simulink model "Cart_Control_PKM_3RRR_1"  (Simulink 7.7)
settings: Solver=FixedStepDiscrete  SolverMode=SingleTasking  StartTime=0  StopTime=6  FixedStep=dt  RelTol=1e-3  SampleTimeConstraint=Specified
InitFcn:
  | % Sampling Times %
  | dt0=0.001; dt1=0.01; samples=10;
  | D2R=pi/180;
undefined symbols (not defined in the file or in its folder): DiscIntNeverNeededParam, Volts
libraries: simulink_extras x4, speedgoatlib_IO311 x3, simulink x3, speedgoatlib x2, xpclib x1

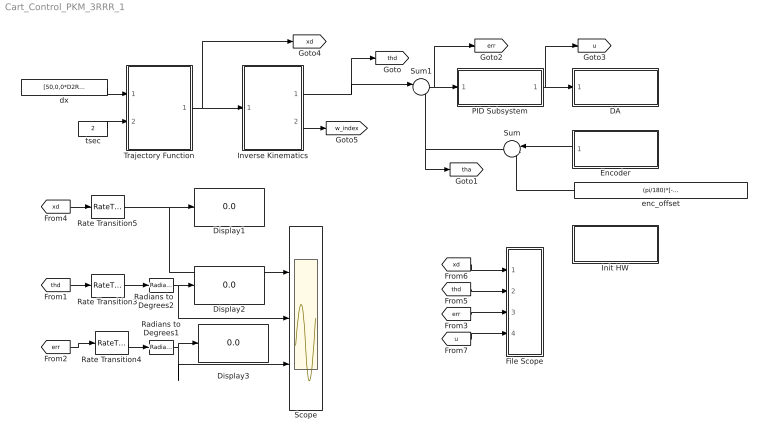
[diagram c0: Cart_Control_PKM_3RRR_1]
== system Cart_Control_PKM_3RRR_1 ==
  DA : Subsystem  TreatAsAtomicUnit=on
  Display1 : Display
  Display2 : Display
  Display3 : Display
  Encoder : Subsystem  TreatAsAtomicUnit=on
  File Scope : Subsystem
  Init HW : Subsystem  TreatAsAtomicUnit=on
  Inverse Kinematics : Stateflow chart  TreatAsAtomicUnit=on
  PID Subsystem : Subsystem  TreatAsAtomicUnit=on
  Radians to Degrees1 : simulink_extras/Transformations/Radians to Degrees  SystemSampleTime=-1
  Radians to Degrees2 : simulink_extras/Transformations/Radians to Degrees  SystemSampleTime=-1
  Rate Transition3 : RateTransition  OutPortSampleTime=dt1
  Rate Transition4 : RateTransition  OutPortSampleTime=dt1
  Rate Transition5 : RateTransition  OutPortSampleTime=dt1
  Scope : Scope  NumInputPorts=3
  Sum : Sum  Inputs=|++
  Sum1 : Sum  Inputs=|+-
  Trajectory Function : Stateflow chart  TreatAsAtomicUnit=on
  dx : Constant  Value=[50,0,0*D2R]'  SampleTime=dt0
  enc_offset : Constant  Value=(pi/180)*[-144.9004,-24.9004,95.0996]'
  tsec : Constant  Value=2  SampleTime=dt0
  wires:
  Sum1/1 -> PID Subsystem/1(In1), [err]
  PID Subsystem/1(Out1) -> [u], DA/1(In1)
  Encoder/1(Out1) -> Sum/1
  enc_offset/1 -> Sum/2
  Sum/1 -> Sum1/2, [tha]
  [xd] -> File Scope/1(xd)
  [thd] -> File Scope/2(thd)
  [err] -> File Scope/3(err)
  [u] -> File Scope/4(u)
  dx/1 -> Trajectory Function/1(dx)
  tsec/1 -> Trajectory Function/2(tsec)
  Trajectory Function/1(xd) -> [xd], Inverse Kinematics/1(xd)
  Inverse Kinematics/1(thd) -> Sum1/1, [thd]
  [thd] -> Rate Transition3/1
  [err] -> Rate Transition4/1
  [xd] -> Rate Transition5/1
  Rate Transition5/1 -> Display1/1, Scope/1
  Rate Transition3/1 -> Radians to Degrees2/1
  Rate Transition4/1 -> Radians to Degrees1/1
  Radians to Degrees2/1 -> Display2/1, Scope/2
  Radians to Degrees1/1 -> Display3/1, Scope/3
  Inverse Kinematics/2(w_index) -> [w_index]

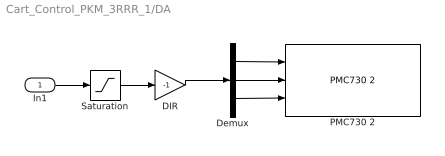
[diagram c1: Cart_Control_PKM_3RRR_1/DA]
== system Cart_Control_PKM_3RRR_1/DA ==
  In1 : Inport
  DIR : Gain  Gain=-1
  Demux : Demux  Outputs=3
  PMC730 2 : speedgoatlib/IO101/PMC730 2  id=1  channel=[1,2,3]  reset=[1,1,1]  initValue=[0,0,0]  ts=dt0  pciSlot=-1
  Saturation : Saturate  UpperLimit=10  LowerLimit=-10
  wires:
  In1/1 -> Saturation/1
  Saturation/1 -> DIR/1
  DIR/1 -> Demux/1
  Demux/1 -> PMC730 2/1
  Demux/2 -> PMC730 2/2
  Demux/3 -> PMC730 2/3

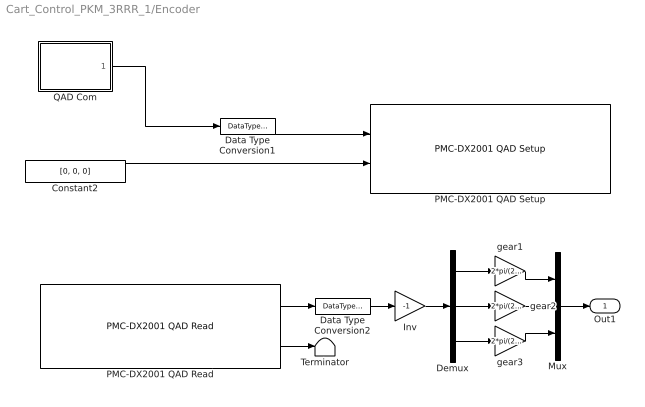
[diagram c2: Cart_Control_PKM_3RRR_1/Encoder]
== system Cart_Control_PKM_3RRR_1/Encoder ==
  Constant2 : Constant  Value=[0, 0, 0]  OutDataTypeStr=Inherit: Inherit via back propagation
  Data Type Conversion1 : DataTypeConversion  OutDataTypeStr=uint8
  Data Type Conversion2 : DataTypeConversion  OutDataTypeStr=double
  Demux : Demux  Outputs=3
  Inv : Gain  Gain=-1
  Mux : Mux  Inputs=3
  PMC-DX2001 QAD Read : speedgoatlib_IO311/PMC-DX2001 QAD Read  id=1  chan=[1, 2, 3]  pciSlot=-1  ts=dt0
  PMC-DX2001 QAD Setup : speedgoatlib_IO311/PMC-DX2001 QAD Setup  id=1  chan=Channel 3 setup  steps1=2000  steps2=2000  steps3=2000  quadrature1=4x  quadrature2=4x  quadrature3=4x  index1=Ignore index input  index2=Ignore index input  index3=Ignore index input  special1=Disabled (cycling counter)  special2=Disabled (cycling counter)  special3=Disabled (cycling counter)  debounce=0  pciSlot=-1  ts=dt0
  QAD Com : Stateflow chart  TreatAsAtomicUnit=on
  Terminator : Terminator
  gear1 : Gain  Gain=2*pi/(23*2000)
  gear2 : Gain  Gain=2*pi/(23*2000)
  gear3 : Gain  Gain=2*pi/(23*2000)
  Out1 : Outport
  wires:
  Constant2/1 -> PMC-DX2001 QAD Setup/2
  PMC-DX2001 QAD Read/2 -> Terminator/1
  PMC-DX2001 QAD Read/1 -> Data Type Conversion2/1
  QAD Com/1(y) -> Data Type Conversion1/1
  Data Type Conversion1/1 -> PMC-DX2001 QAD Setup/1
  Data Type Conversion2/1 -> Inv/1
  Mux/1 -> Out1/1
  Demux/1 -> gear1/1
  gear1/1 -> Mux/1
  Demux/2 -> gear2/1
  gear2/1 -> Mux/2
  Inv/1 -> Demux/1
  Demux/3 -> gear3/1
  gear3/1 -> Mux/3

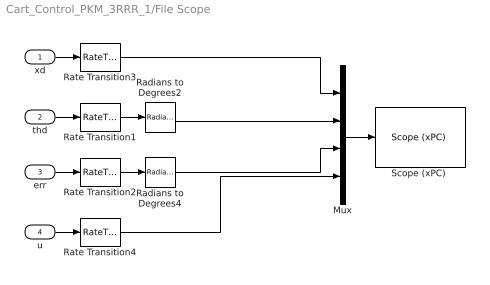
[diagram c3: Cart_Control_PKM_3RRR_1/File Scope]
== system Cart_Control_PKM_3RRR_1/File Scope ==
  xd : Inport
  thd : Inport  Port=2
  err : Inport  Port=3
  u : Inport  Port=4
  Mux : Mux
  Radians to Degrees2 : simulink_extras/Transformations/Radians to Degrees  SystemSampleTime=-1
  Radians to Degrees4 : simulink_extras/Transformations/Radians to Degrees  SystemSampleTime=-1
  Rate Transition{1..4} (4 alike) : RateTransition  OutPortSampleTime=dt1
  "Scope (xPC) " : xpclib/Misc./Scope (xPC)   SystemSampleTime=-1  scopeno=1  scopetype=File  autostart=on  viewmode=Graphical redraw  formatstr='%15.6f'  grid=on  ylimits=[0,0]  nosamples=100  noprepostsamples=0  interleave=1  triggermode=FreeRun  triggersignal=1  triggerlevel=0.0  triggerslope=Either  triggerscope=1  triggersample=0  filename=step2.dat  mode=Lazy  writesize=512  autorestart=on  dynamicfilemode=off  maxwritefilesize=512*1024^2
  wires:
  Radians to Degrees2/1 -> Mux/2
  Radians to Degrees4/1 -> Mux/3
  Rate Transition1/1 -> Radians to Degrees2/1
  Rate Transition2/1 -> Radians to Degrees4/1
  thd/1 -> Rate Transition1/1
  err/1 -> Rate Transition2/1
  Rate Transition3/1 -> Mux/1
  xd/1 -> Rate Transition3/1
  u/1 -> Rate Transition4/1
  Mux/1 -> "Scope (xPC) "/1
  Rate Transition4/1 -> Mux/4

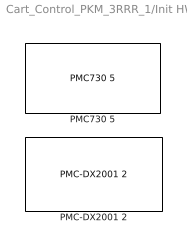
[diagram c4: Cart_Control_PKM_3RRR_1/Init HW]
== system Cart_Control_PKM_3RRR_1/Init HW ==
  PMC-DX2001 2 : speedgoatlib_IO311/PMC-DX2001 2  id=1  fpga1=IO311_3PWM_3CAP_3QAD_INT.fpga  fpga2=PWM_Triangle_DX501.fpga  fpga3=PWM_Triangle_DX501.fpga  fpga4=PWM_Triangle_DX501.fpga  fpga5=PWM_Triangle_DX501.fpga  fpga6=PWM_Triangle_DX501.fpga  fpga7=PWM_Triangle_DX501.fpga  fpga8=PWM_Triangle_DX501.fpga  fpga9=PWM_Triangle_DX501.fpga  fpga10=PWM_Triangle_DX501.fpga  group=Module setup  pciSlot=-1  lowerDirection=[ones(1,5), zeros(1, 7), ones(1, 1), ones(1, 3)]  lowerReset=[1]  lowerValue=[0]  upperDirection=[ones(1, 8), zeros(1, 8)]  upperReset=[1]  upperValue=[0]
  PMC730 5 : speedgoatlib/IO101/PMC730 5  id=1  group=Analog output setup  pciSlot=-1  adStartChannel=1  adNumChannel=1  adCoupling=Single-ended  adRange=-10 .. 10 Volts  adAcqMode=Standard  daChannel=[1,2, 3]  daReset=[1,1, 1]  daInitValue=[0,0,0]  diChannel=[1]  diDebounce=[0]  doChannel=[1]  doReset=[1]  doInitValue=[0]

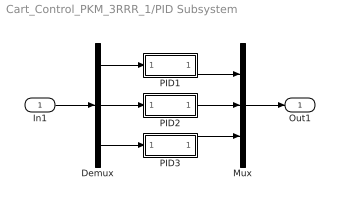
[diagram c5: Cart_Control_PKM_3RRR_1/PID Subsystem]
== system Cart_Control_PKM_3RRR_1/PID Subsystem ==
  In1 : Inport
  Demux : Demux  Outputs=3
  Mux : Mux  Inputs=3
  PID1 : Subsystem
  PID2 : Subsystem
  PID3 : Subsystem
  Out1 : Outport
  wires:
  In1/1 -> Demux/1
  Demux/1 -> PID1/1(In1)
  PID1/1(Out1) -> Mux/1
  Demux/2 -> PID2/1(In1)
  PID2/1(Out1) -> Mux/2
  Mux/1 -> Out1/1
  Demux/3 -> PID3/1(In1)
  PID3/1(Out1) -> Mux/3

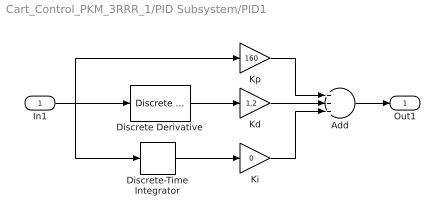
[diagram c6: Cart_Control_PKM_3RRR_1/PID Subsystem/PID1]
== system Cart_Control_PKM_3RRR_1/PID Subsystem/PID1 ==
  In1 : Inport
  Add : Sum  Inputs=+++
  Discrete Derivative : simulink/Discrete/Discrete Derivative  SystemSampleTime=-1  gainval=1.0  ICPrevScaledInput=0.0  OutMin=[]  OutMax=[]  OutDataType=fixdt(1, 16)  OutScaling=2^-10  DoSatur=off
  Discrete-Time Integrator : DiscreteIntegrator  SampleTime=dt0  ICPrevOutput=DiscIntNeverNeededParam  ICPrevScaledInput=DiscIntNeverNeededParam
  Kd : Gain  Gain=1.2
  Ki : Gain  Gain=0
  Kp : Gain  Gain=160
  Out1 : Outport
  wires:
  Discrete-Time Integrator/1 -> Ki/1
  Kp/1 -> Add/1
  Kd/1 -> Add/2
  Ki/1 -> Add/3
  Discrete Derivative/1 -> Kd/1
  Add/1 -> Out1/1
  In1/1 -> Kp/1, Discrete Derivative/1, Discrete-Time Integrator/1

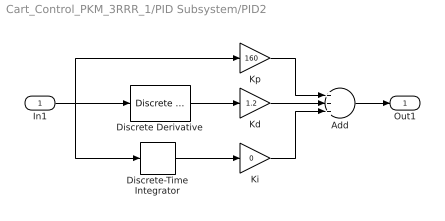
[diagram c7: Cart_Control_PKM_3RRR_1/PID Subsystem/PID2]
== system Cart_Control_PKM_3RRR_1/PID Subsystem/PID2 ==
  In1 : Inport
  Add : Sum  Inputs=+++
  Discrete Derivative : simulink/Discrete/Discrete Derivative  SystemSampleTime=-1  gainval=1.0  ICPrevScaledInput=0.0  OutMin=[]  OutMax=[]  OutDataType=fixdt(1, 16)  OutScaling=2^-10  DoSatur=off
  Discrete-Time Integrator : DiscreteIntegrator  SampleTime=dt0  ICPrevOutput=DiscIntNeverNeededParam  ICPrevScaledInput=DiscIntNeverNeededParam
  Kd : Gain  Gain=1.2
  Ki : Gain  Gain=0
  Kp : Gain  Gain=160
  Out1 : Outport
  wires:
  Discrete-Time Integrator/1 -> Ki/1
  Kp/1 -> Add/1
  Kd/1 -> Add/2
  Ki/1 -> Add/3
  Discrete Derivative/1 -> Kd/1
  Add/1 -> Out1/1
  In1/1 -> Kp/1, Discrete Derivative/1, Discrete-Time Integrator/1

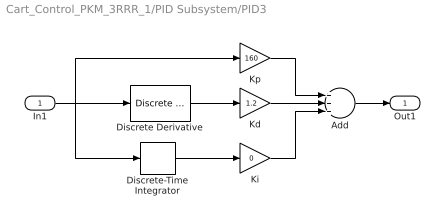
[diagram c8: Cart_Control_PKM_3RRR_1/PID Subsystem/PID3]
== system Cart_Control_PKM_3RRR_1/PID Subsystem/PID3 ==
  In1 : Inport
  Add : Sum  Inputs=+++
  Discrete Derivative : simulink/Discrete/Discrete Derivative  SystemSampleTime=-1  gainval=1.0  ICPrevScaledInput=0.0  OutMin=[]  OutMax=[]  OutDataType=fixdt(1, 16)  OutScaling=2^-10  DoSatur=off
  Discrete-Time Integrator : DiscreteIntegrator  SampleTime=dt0  ICPrevOutput=DiscIntNeverNeededParam  ICPrevScaledInput=DiscIntNeverNeededParam
  Kd : Gain  Gain=1.2
  Ki : Gain  Gain=0
  Kp : Gain  Gain=160
  Out1 : Outport
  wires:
  Discrete-Time Integrator/1 -> Ki/1
  Kp/1 -> Add/1
  Kd/1 -> Add/2
  Ki/1 -> Add/3
  Discrete Derivative/1 -> Kd/1
  Add/1 -> Out1/1
  In1/1 -> Kp/1, Discrete Derivative/1, Discrete-Time Integrator/1

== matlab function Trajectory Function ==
function xd = fcn(dx, tsec)

persistent index xd_p

MAX_CH=3;       % 3 Actuators %
dt=0.001;       % Step time is 10 msec %

% Initializing Variables %
if isempty(index), index=0; end
if isempty(xd_p), xd_p=zeros(MAX_CH,1); end
xd=zeros(MAX_CH,1);
x0=[0,0,0]';

tout=index*dt;
if index<(tsec/dt)
    [c] = coeff_3rd(x0, zeros(MAX_CH,1), x0+dx, zeros(MAX_CH,1), tsec);
    for ch=1:MAX_CH
        xd(ch,1)=c(ch,1)+c(ch,2)*tout+c(ch,3)*tout^2+c(ch,4)*tout^3;    
    end
    xd_p=xd;
else
    xd=xd_p;
end
index=index+1;

function [c] = coeff_3rd(sp, sv, ep, ev, tsec)
MAX_CH=3;
c=zeros(MAX_CH,4);
for ch=1:MAX_CH
    c(ch,1)=sp(ch,1);
    c(ch,2)=sv(ch,1);
    c(ch,3)=(3.0*(ep(ch,1)-sp(ch,1))-(2.0*sv(ch,1)+ev(ch,1))*tsec)/(tsec*tsec);
    c(ch,4)=(-2.0*(ep(ch,1)-sp(ch,1))+(sv(ch,1)+ev(ch,1))*tsec)/(tsec*tsec*tsec);
end

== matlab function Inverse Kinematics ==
function [thd,w_index]  = fcn(xd)

persistent index thd_p

% Initializing Variables %
if isempty(index), index=0; end
if isempty(thd_p), thd_p=(pi/180)*[-144.9004,-24.9004,95.0996]'; end

% Kinematic Parameters %
ra=150; rb=35; L1=100; L2=100;

pos=xd(1:2,1); ang=xd(3,1);

w_index=1;  % In workspace %

% Vertex Points %
A=ra*[0,-sqrt(3)/2, +sqrt(3)/2; 1, -1/2, -1/2];
B=rb*[0,-sqrt(3)/2, +sqrt(3)/2; 1, -1/2, -1/2];

th=zeros(3,1);
R=[cos(ang), -sin(ang); sin(ang), cos(ang)];
for i=1:3
    d=pos+R*B(:,i)-A(:,i);
    e1=-2*L1*d(2,1); e2=-2*L1*d(1,1);
    e3=d(1,1)^2+d(2,1)^2+L1^2-L2^2;
    temp=e1^2+e2^2-e3^2;
    if temp>=0
        th(i,1)=2*atan((-e1-sqrt(temp))/(e3-e2));
    else
        th(i,1)=0;
        w_index=-1;
        %disp('Out of Workspace');
    end
end

% Result %
if w_index==1
    thd=[th(1,1), th(2,1), th(3,1)]';
else
    thd=thd_p;
end

% Save the current value %
thd_p=thd;

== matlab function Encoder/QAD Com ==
function y = fcn()

persistent index

if isempty(index), index=0; end

if index==0
    y=[1,1,1];      %  Reset %
else
    y = [0,0,0];
end

index=index+1;
